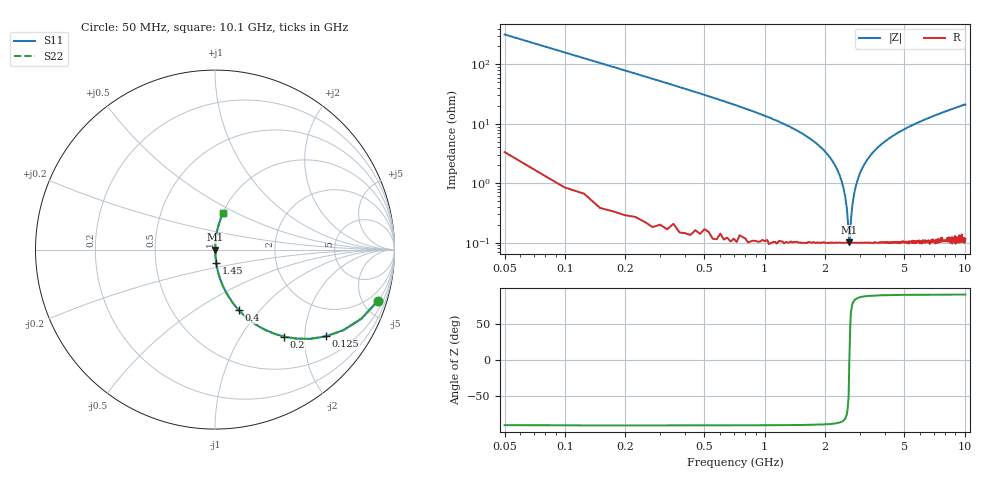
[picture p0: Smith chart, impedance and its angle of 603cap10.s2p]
! AVX Thin Film Operation		Date: November 2004
! Description: Accu-P® Series, Thin Film, SMD, RF Capacitor
! Part Number: 06035J100FBT
! 50 MHz  -  10.05 GHz
! Serial Measurements
# hz S db R 50
!	S11		S21		S12		S22
!	dB	Phase	dB	Phase	dB	Phase	dB	Phase
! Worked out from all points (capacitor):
!   400 points, 50 MHz to 10.1 GHz, reference 50 ohm
!   read as one part in series: C = 10 pF near 100 MHz
!   lowest |Z| = 101 mohm at 2.65 GHz (marker M1)
!   series resonance near 2.653 GHz, so ESL is about 360 pH
!   S11 on the Smith chart (normalised r, x): 50 MHz: 1.07, -6.36; 125 MHz: 1.01, -2.54; 200 MHz: 1.01, -1.58; 400 MHz: 1.00, -0.78; 1.45 GHz: 1.00, -0.15; 10.1 GHz: 1.00, +0.42
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5e7  -0.44 -17.4  -10.50 72.0  -10.50 72.0  -0.44 -17.4
7.5e7  -0.90 -25.2  -7.43 64.4  -7.43 64.4  -0.90 -25.2
1.25e8  -2.12 -38.1  -4.19 51.6  -4.19 51.6  -2.12 -38.1
2e8  -4.16 -51.5  -2.13 38.3  -2.13 38.3  -4.16 -51.5
4e8  -8.83 -68.6  -0.62 21.2  -0.62 21.2  -8.83 -68.6
8e8  -15.00 -79.4  -0.15 10.2  -0.15 10.2  -15.00 -79.4
1.45e9  -22.30 -84.8  -0.03 4.4  -0.03 4.4  -22.30 -84.8
1.73e9  -25.50 -85.9  -0.02 3.0  -0.02 3.0  -25.50 -85.9
2.13e9  -31.40 -86.3  -0.01 1.5  -0.01 1.5  -31.40 -86.3
2.43e9  -39.30 -84.1  -0.01 0.6  -0.01 0.6  -39.30 -84.1
2.53e9  -44.40 -80.1  -0.01 0.3  -0.01 0.3  -44.40 -80.1
2.58e9  -48.60 -74.1  -0.01 0.2  -0.01 0.2  -48.60 -74.1
2.65e9  -59.90 -6.7  -0.01 0.0  -0.01 0.0  -59.90 -6.7
2.75e9  -47.10 76.7  -0.01 -0.2  -0.01 -0.2  -47.10 76.7
2.85e9  -41.20 82.9  -0.01 -0.5  -0.01 -0.5  -41.20 82.9
3.1e9  -34.50 85.9  -0.01 -1.1  -0.01 -1.1  -34.50 85.9
3.4e9  -30.40 86.4  -0.01 -1.7  -0.01 -1.7  -30.40 86.4
4.05e9  -25.60 85.9  -0.02 -3.0  -0.02 -3.0  -25.60 85.9
5.08e9  -21.60 84.5  -0.04 -4.8  -0.04 -4.8  -21.60 84.5
6.75e9  -17.90 82.2  -0.08 -7.3  -0.08 -7.3  -17.90 82.2
8.43e9  -15.40 79.9  -0.14 -9.7  -0.14 -9.7  -15.40 79.9
1.01e10  -13.70 77.8  -0.20 -11.9  -0.20 -11.9  -13.70 77.8
